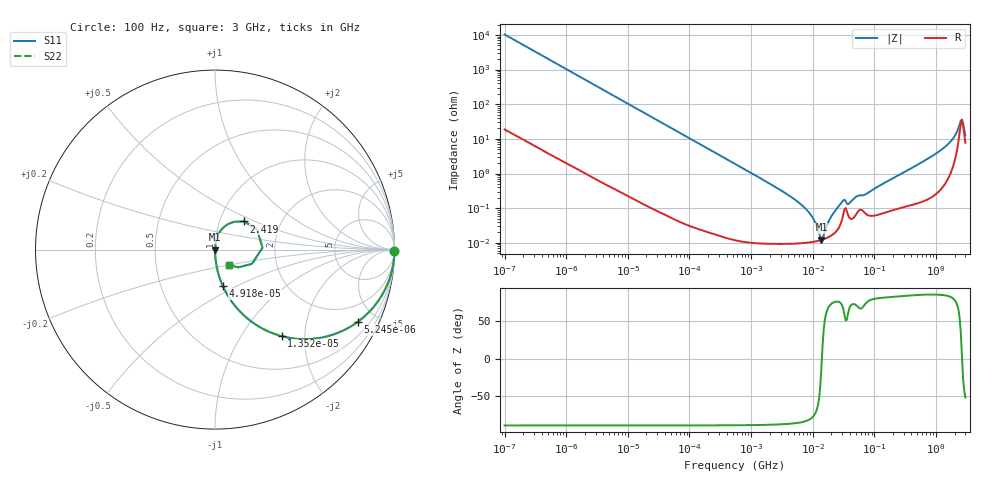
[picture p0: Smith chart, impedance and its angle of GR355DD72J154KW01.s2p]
!Murata Part Number: GR355DD72J154KW01
!These Parameters are Measured in Series Mode Connection
!Data Generated on Mar 13, 2026
!  o--ll--o
!Port1  Port2
!  o------o
!Operation Temp=25[degC], DC Bias Voltage=0[V]
!Freq. Start=100[Hz] Stop=3[GHz] 401[Steps]
# Hz S RI R 50
!Freq.(Hz) S11(Real) S11(Imag) S21(Real) S21(Imag) S12(Real) S12(Imag) S22(Real) S22(Imag)
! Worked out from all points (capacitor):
!   401 points, 100 Hz to 3 GHz, reference 50 ohm
!   read as one part in series: C = 154 nF near 109 Hz
!   lowest |Z| = 12.4 mohm at 13.82 MHz (marker M1)
!   series resonance near 14.07 MHz, so ESL is about 830 pH
!   S11 on the Smith chart (normalised r, x): 100 Hz: open; 5.245 kHz: 1.01, -3.95; 13.52 kHz: 1.00, -1.53; 49.18 kHz: 1.00, -0.42; 2.419 GHz: 1.30, +0.43; 3 GHz: 1.15, -0.20
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100  0.9999 -0.0097  0.000112 0.0097  0.000112 0.0097  0.9999 -0.0097
1788  0.9707 -0.1677  0.0293 0.1677  0.0293 0.1677  0.9707 -0.1677
5245  0.7955 -0.4023  0.2045 0.4023  0.2045 0.4023  0.7955 -0.4023
13520  0.3709 -0.4819  0.6291 0.4819  0.6291 0.4819  0.3709 -0.4819
31977  0.096 -0.2934  0.904 0.2934  0.904 0.2934  0.096 -0.2934
49177  0.0432 -0.2021  0.9568 0.2021  0.9568 0.2021  0.0432 -0.2021
547723  0.00048 -0.019  0.9995 0.019  0.9995 0.019  0.00048 -0.019
4513443  9.84e-05 -0.00208  0.9999 0.00208  0.9999 0.00208  9.84e-05 -0.00208
7246509  9.99e-05 -0.00106  0.9999 0.00106  0.9999 0.00106  9.99e-05 -0.00106
9794414  0.000106 -0.000553  0.9999 0.000553  0.9999 0.000553  0.000106 -0.000553
1.382041e7  0.000121 -2.67e-05  0.9999 2.67e-05  0.9999 2.67e-05  0.000121 -2.67e-05
1.506283e7  0.000128 0.000104  0.9999 -0.000104  0.9999 -0.000104  0.000128 0.000104
2.035898e7  0.000166 0.000587  0.9998 -0.000587  0.9998 -0.000587  0.000166 0.000587
2.999103e7  0.000484 0.00145  0.9995 -0.00145  0.9995 -0.00145  0.000484 0.00145
3.882828e7  0.000547 0.00125  0.9995 -0.00125  0.9995 -0.00125  0.000547 0.00125
5.248048e7  0.000736 0.00209  0.9993 -0.00209  0.9993 -0.00209  0.000736 0.00209
1.751444e8  0.000853 0.00636  0.9991 -0.00636  0.9991 -0.00636  0.000853 0.00636
1.268426e9  0.00646 0.0504  0.9935 -0.0504  0.9935 -0.0504  0.00646 0.0504
1.868531e9  0.0239 0.0944  0.9761 -0.0944  0.9761 -0.0944  0.0239 0.0944
2.419119e9  0.1604 0.1569  0.8396 -0.1569  0.8396 -0.1569  0.1604 0.1569
2.636591e9  0.2648 0.0106  0.7352 -0.0106  0.7352 -0.0106  0.2648 0.0106
3e9  0.0798 -0.0858  0.9202 0.0858  0.9202 0.0858  0.0798 -0.0858
